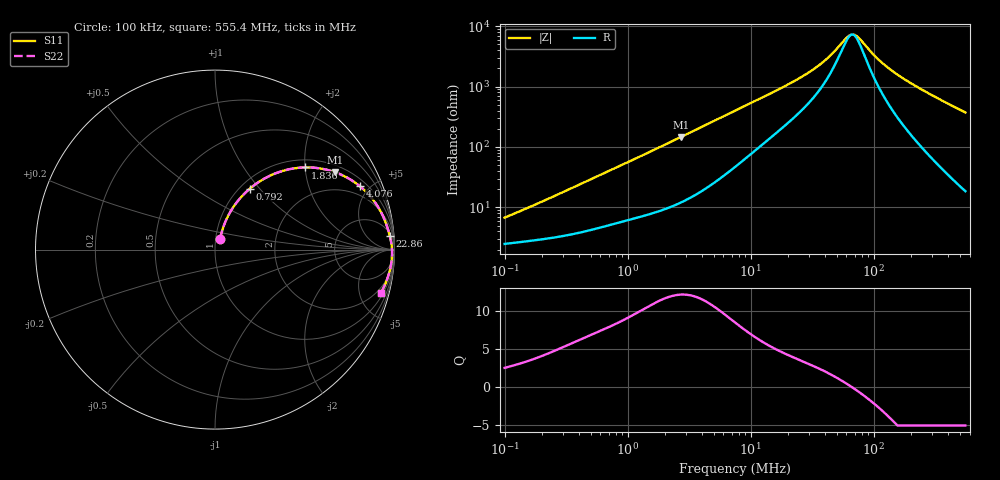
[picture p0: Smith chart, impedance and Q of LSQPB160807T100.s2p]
! LSQPB160807T100  S-PARAMETER MODEL  ( General Type )
! Model Generated by TAIYO YUDEN Corporation (http://www.ty-top.com)
! Version 1.0
! TAIYO YUDEN Control No. 110308NG25SB-FKC
! Copyright(c) 2011 TAIYO YUDEN CO.,LTD. All Rights Reserved.
! Product Description (link to TY-COMPAS)
! https://ds.yuden.co.jp/TYCOMPAS/or/detail?pn=LSQPB160807T100M&u=M
! Products Name : Inductors
! Characteristics :
!  Inductance : 10 uH , SRF(min) : 45 MHz , DC Resistance(max) : 2.6 Ohm
!  Rated Current : Saturation :170 mA , Temp Rise : 220 mA (40 degC)
!  Case Size : 1.6 x 0.8 / 0.063 x 0.031 [mm/inch] , Thickness : 0.7 / 0.028 [mm/inch]
!  (Conditions: Temperature = 25 degC , DC Bias Current/Voltage = 0A / 0V)
! External Node Assignments :
!  1  o---GGG---o  2
! GND o---------o GND
! Frequency Range : 0.1MHz  -  555.443392MHz  [ 402 STEP ]
# MHz S RI R 50
! Freq[MHz].  S11 Real  S11 Imag  S21 Real  S21 Imag  S12 Real  S12 Imag  S22 Real  S22 Imag
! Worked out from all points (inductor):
!   401 points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, 100 kHz to 555.4 MHz, reference 50 ohm
!   read as one part in series: L = 9.72 uH near 129.5 kHz
!   highest Q = 12.1 at 2.706 MHz (marker M1), where L = 8.59 uH
!   self-resonance near 66.65 MHz
!   S11 on the Smith chart (normalised r, x): 100 kHz: 1.05, +0.13; 792 kHz: 1.11, +0.89; 1.836 MHz: 1.18, +2.00; 4.076 MHz: 1.38, +4.37; 22.86 MHz: 7, +24; 555.4 MHz: 1.37, -7.44
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0.1  0.028 0.0598  0.972 -0.0598  0.972 -0.0598  0.028 0.0598
0.212645  0.044 0.1186  0.956 -0.1186  0.956 -0.1186  0.044 0.1186
0.423865  0.0887 0.2161  0.9113 -0.2161  0.9113 -0.2161  0.0887 0.2161
0.791979  0.1952 0.3403  0.8048 -0.3403  0.8048 -0.3403  0.1952 0.3403
1.167407  0.3135 0.415  0.6865 -0.415  0.6865 -0.415  0.3135 0.415
1.796612  0.4915 0.4576  0.5085 -0.4576  0.5085 -0.4576  0.4915 0.4576
1.83576  0.5011 0.4579  0.4989 -0.4579  0.4989 -0.4579  0.5011 0.4579
2.705981  0.6692 0.431  0.3308 -0.431  0.3308 -0.431  0.6692 0.431
4.075633  0.8078 0.3528  0.1922 -0.3528  0.1922 -0.3528  0.8078 0.3528
5.511344  0.875 0.2849  0.125 -0.2849  0.125 -0.2849  0.875 0.2849
7.615203  0.92 0.218  0.08 -0.218  0.08 -0.218  0.92 0.218
12.77497  0.9566 0.1353  0.0434 -0.1353  0.0434 -0.1353  0.9566 0.1353
22.86247  0.9746 0.0738  0.0254 -0.0738  0.0254 -0.0738  0.9746 0.0738
31.58981  0.9802 0.0486  0.0198 -0.0486  0.0198 -0.0486  0.9802 0.0486
42.71786  0.9837 0.028  0.0163 -0.028  0.0163 -0.028  0.9837 0.028
60.31079  0.9861 0.00622  0.0139 -0.00622  0.0139 -0.00622  0.9861 0.00622
67.17428  0.9865 -0.000486  0.0135 0.000486  0.0135 0.000486  0.9865 -0.000486
74.81885  0.9867 -0.00726  0.0133 0.00726  0.0133 0.00726  0.9867 -0.00726
103.3796  0.9866 -0.0286  0.0134 0.0286  0.0134 0.0286  0.9866 -0.0286
133.898  0.9854 -0.0478  0.0146 0.0478  0.0146 0.0478  0.9854 -0.0478
239.6279  0.9767 -0.1043  0.0233 0.1043  0.0233 0.1043  0.9767 -0.1043
555.4434  0.9223 -0.244  0.0777 0.244  0.0777 0.244  0.9223 -0.244
